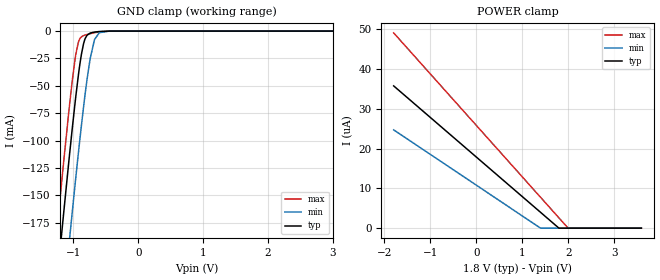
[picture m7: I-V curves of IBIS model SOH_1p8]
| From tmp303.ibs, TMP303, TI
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|   Model
[Model]   SOH_1p8
Model_type   Input
Vinl = 0.54
Vinh = 1.26
|   typ   min   max
C_comp   1pF   1pF   1pF
[Voltage Range]   1.8   1.4   2
[Temperature Range]   25   125   -40
[Power Clamp Reference]   1.8   1.4   2
[GND Clamp Reference]   -0   -0   -0
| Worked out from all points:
|   GND clamp passes 1 mA (typ) near -0.68 V on its own axis
[GND Clamp]
|   Voltage   I(typ)   I(min)   I(max)
-1.8V     -577.8mA   -655.1mA   -532mA
-1.433V   -342mA     -420.5mA   -295.2mA
-1.217V   -206.8mA   -285.4mA   -159.7mA
-1.184V   -186.9mA   -265.4mA   -139.9mA
-1.066V   -116.1mA   -193.5mA   -70.51mA
-963mV    -59.55mA   -133.7mA   -21.17mA
-876.6mV  -21.18mA   -86.19mA   -5.212mA
-817.2mV  -6.601mA   -56.42mA   -3.574mA
-741.6mV  -1.821mA   -25.03mA   -2.386mA
-676.8mV  -929.8uA   -8.278mA   -1.522mA
-601.2mV  -386.3uA   -1.494mA   -704.6uA
3.595V    0A         0A         0A
[POWER Clamp]
|   Voltage   I(typ)   I(min)   I(max)
-1.8V     35.75uA    24.7uA     49.06uA
1.397V    3.999uA    19.11nA    7.783uA
1.796V    30.22nA    0A         2.623uA
1.996V    0A         0A         43.59nA
3.595V    0A         0A         0A
